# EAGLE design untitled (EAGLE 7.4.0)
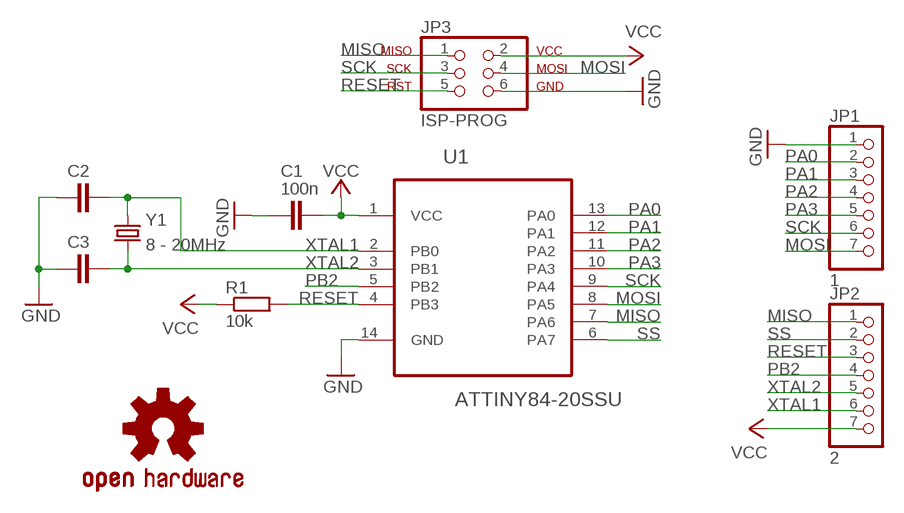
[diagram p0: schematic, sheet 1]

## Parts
C1  100n  CAP805  [0805]
C2  CAP805  [0805]
C3  CAP805  [0805]
JP1  1  PINHD-1X7  [1X07]
JP2  2  PINHD-1X7  [1X07]
JP3  ISP-PROG  PINHD-2X3_ISP_2.54  [2X03]
LOGO2  OSHW-LOGOS  [OSHW-LOGO-S]
R1  10k  RES805  [0805]
U1  ATTINY84-20SSU  [SOIC127P600X175-14N]
Y1  8 - 20MHz  CRYSTALTXC-7A  [CRYSTAL-TXC-7A]

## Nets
GND: C1.2 C2.2 C3.2 JP1.1 JP3.6 U1.14(GND)
MISO: JP2.1 JP3.1 U1.7(PA6)
MOSI: JP1.7 JP3.4 U1.8(PA5)
PA0: JP1.2 U1.13(PA0)
PA1: JP1.3 U1.12(PA1)
PA2: JP1.4 U1.11(PA2)
PA3: JP1.5 U1.10(PA3)
PB2: JP2.4 U1.5(PB2)
RESET: JP2.3 JP3.5 R1.2 U1.4(PB3)
SCK: JP1.6 JP3.3 U1.9(PA4)
SS: JP2.2 U1.6(PA7)
VCC: C1.1 JP2.7 JP3.2 R1.1 U1.1(VCC)
XTAL1: C2.1 JP2.6 U1.2(PB0) Y1.P$1
XTAL2: C3.1 JP2.5 U1.3(PB1) Y1.P$2

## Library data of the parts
C1-C3 = _ssr:CAP805
JP1 JP2 = pinhead:PINHD-1X7: PIN HEADER
JP3 = _ssr:PINHD-2X3_ISP: PIN HEADER
LOGO2 = SparkFun-Aesthetics:OSHW-LOGO: Open Source Hardware Logo
R1 = _ssr:RES805
U1 = Atmel_By_element14_Batch_1-00:ATTINY84-20SSU: 8-bit Microcontroller with Bytes In-System Programmable Flash; MPN: ATTINY84-20SSU; OC_FARNELL: 1636955; OC_NEWARK: 03P2040; PACKAGE: SOIC-14; SUPPLIER: Atmel
Y1 = SparkFun-FreqCtrl:CRYSTAL: Various standard crystals. Proven footprints.

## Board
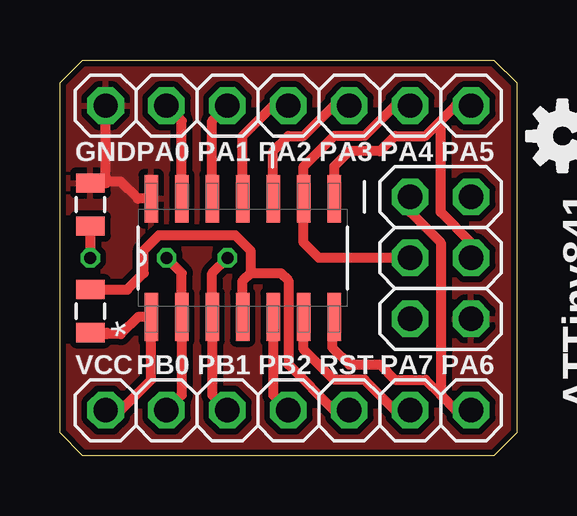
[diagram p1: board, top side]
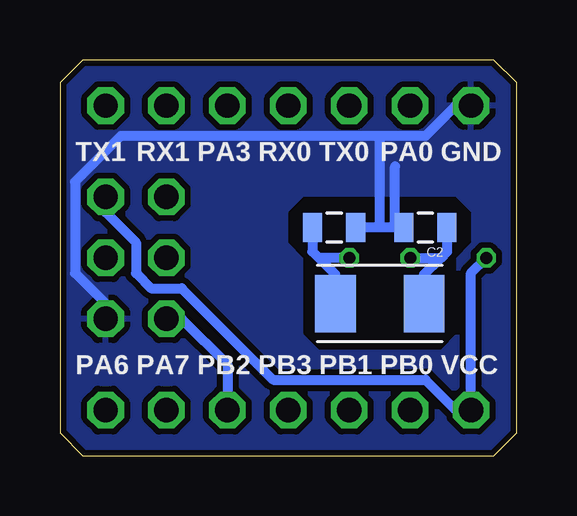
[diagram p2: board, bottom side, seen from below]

Size 19.05 x 16.51 mm. Coordinates in mm from the lower left corner, seen from the top.
Outline: 0.95,16.51 18.1,16.51 19.05,15.56 19.05,0.95 18.1,0 0.95,0 0,0.95 0,15.56 0.95,16.51
Copper layers (1*16): Top 0.035mm / dielectric 1.5mm / Bottom 0.035mm
Design rules "Elecrow_2-layer_eagle_rule": minimum track width 6mil, minimum drill 12mil, track to track 6mil, track to pad 6mil, pad to pad 6mil, via to via 6mil, smd to smd 0mil, copper to edge 10mil, drill to drill 10mil, minimum pad ring 10mil, minimum via ring 6mil, stop-mask expansion 2mil, vias tented up to drill 100mil, thermal gap 10mil

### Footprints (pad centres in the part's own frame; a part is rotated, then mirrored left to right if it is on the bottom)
0805 = smd 0.8 x 1.2: 1 -0.9,0; 2 0.9,0
1X07 = drill 1.016 octagon: 1 -7.62,0; 2 -5.08,0; 3 -2.54,0; 4 0,0; 5 2.54,0; 6 5.08,0; 7 7.62,0
2X03 = drill 1.016 octagon: 1 -2.54,-1.27; 2 -2.54,1.27; 3 0,-1.27; 4 0,1.27; 5 2.54,-1.27; 6 2.54,1.27
SOIC127P600X175-14N = smd 1.981 x 0.559: 1 -2.464,3.81; 2 -2.464,2.54; 3 -2.464,1.27; 4 -2.464,0; 5 -2.464,-1.27; 6 -2.464,-2.54; 7 -2.464,-3.81; 8 2.464,-3.81; 9 2.464,-2.54; 10 2.464,-1.27; 11 2.464,0; 12 2.464,1.27; 13 2.464,2.54; 14 2.464,3.81
CRYSTAL-TXC-7A = smd 1.7 x 2.4: P$1 1.85,0; P$2 -1.85,0

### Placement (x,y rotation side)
C1  1.27,10.48 90 top
C2  3.81,9.53 180 bottom
C3  7.62,9.53 0 bottom
JP1  9.53,14.61 0 top
JP2  9.53,1.91 180 top
JP3  15.88,8.26 270 top
LOGO2  20.95,13.34 90 top
R1  1.27,6.03 90 top
U1  7.62,8.26 90 top
Y1  5.71,6.35 0 bottom

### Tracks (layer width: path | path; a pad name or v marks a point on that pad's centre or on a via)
GND
  Top 0.406: 1.96,11.38 C1.2 1.96,11.43 | 1.96,11.43 2.54,11.43 3.25,10.72 U1.14 | 1.96,11.43 1.91,11.43 JP1.1
  Bottom 0.406: 2.54,14.61 3.81,13.34 5.71,13.34 | 5.71,13.34 16.51,13.34 18.41,11.43 18.41,7.62 17.14,6.35 JP3.6 | 5.71,9.53 C3.2 | C2.2 5.08,9.53 | 5.08,9.53 5.71,9.53 | 5.71,9.53 5.71,13.34 | 5.08,9.53 5.08,12.06
  pour Bottom (isolate 0.254): 0,16.51 0,0 19.05,0 19.05,16.51
  cutout Bottom: 1.91,10.16 1.91,8.89 2.54,8.26 2.54,5.08 3.17,4.45 8.26,4.45 8.89,5.08 8.89,8.26 9.53,8.89 9.53,10.16 8.89,10.79 2.54,10.79
  pour Top (isolate 0.254): 0,16.51 19.05,16.51 19.05,0 0,0
MISO
  Top 0.406: JP3.1 14.61,10.16 15.88,8.89 15.88,2.54 | U1.7 11.35,5.79 11.35,4.52 12.06,3.81 13.34,3.81 13.97,3.17 15.24,3.17 15.88,2.54 | JP2.1 16.51,1.91 15.88,2.54
MOSI
  Top 0.406: JP3.4 17.14,8.89 15.88,10.16 15.88,13.97 | JP1.7 16.51,14.61 15.88,13.97 | 11.35,10.72 U1.8 11.43,12.06 12.06,12.7 13.34,12.7 13.97,13.34 15.24,13.34 15.88,13.97
PA0
  Top 0.406: U1.13 5.08,13.97 JP1.2
PA1
  Top 0.406: U1.12 6.35,13.97 JP1.3
PA2
  Top 0.406: U1.11 7.62,13.34 8.89,14.61 JP1.4
PA3
  Top 0.406: U1.10 8.89,12.7 9.53,13.34 10.16,13.34 11.43,14.61 JP1.5
PB2
  Top 0.406: U1.5 8.89,2.54 JP2.4
RESET
  Top 0.406: 1.85,6.93 R1.2 2.81,6.93 3.49,7.62 3.49,8.57 4.13,9.21 7.3,9.21 7.94,8.57 7.94,7.62 | JP2.3 11.43,1.91 9.53,3.81 9.53,7.3 9.21,7.62 7.94,7.62 | U1.4 7.62,7.3 7.94,7.62
  Bottom 0.406: JP3.5 13.97,5.71 12.06,3.81 JP2.3
SCK
  Top 0.406: JP1.6 13.97,14.61 12.7,13.34 11.43,13.34 10.16,12.06 U1.9 10.16,8.89 10.79,8.26 JP3.3
SS
  Top 0.406: JP2.2 13.97,1.91 12.7,3.17 11.43,3.17 10.16,4.45 U1.6
VCC  (via drill 0.5)
  Top 0.406: JP2.7 2.54,1.91 3.81,3.17 U1.1 3.25,5.79 2.54,5.08 1.96,5.08 R1.1 1.96,5.13 1.91,5.08 | C1.1 v1.27,8.26
  Bottom 0.406: v1.27,8.26 1.91,7.62 JP2.7 2.54,1.91 3.81,3.17 10.16,3.17 13.97,6.99 15.24,6.99 15.88,7.62 15.88,8.89 17.14,10.16 JP3.2
XTAL1  (via drill 0.5)
  Top 0.406: JP2.6 5.08,2.54 U1.2 5.08,7.62 v4.45,8.26
  Bottom 0.406: C2.1 2.91,8.52 3.17,8.26 | Y1.P$1 3.87,7.57 3.17,8.26 | v4.45,8.26 3.17,8.26
XTAL2  (via drill 0.5)
  Top 0.406: JP2.5 6.35,2.54 U1.3 6.35,7.62 v6.99,8.26
  Bottom 0.406: C3.1 8.52,8.52 8.26,8.26 | Y1.P$2 7.57,7.57 8.26,8.26 | v6.99,8.26 8.26,8.26

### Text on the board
tPlace: GND | PA0 | PA1 | PA2 | PA3 | PA4 | PA5 | VCC | PB0 | PB1 | PB2 | RST | PA7 | PA6 | ATTiny841 | sschultewolter | 10-2015
bPlace: GND | PA0 | TX0 | RX0 | PA3 | RX1 | TX1 | VCC | PB0 | PB1 | PB3 | PB2 | PA7 | PA6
